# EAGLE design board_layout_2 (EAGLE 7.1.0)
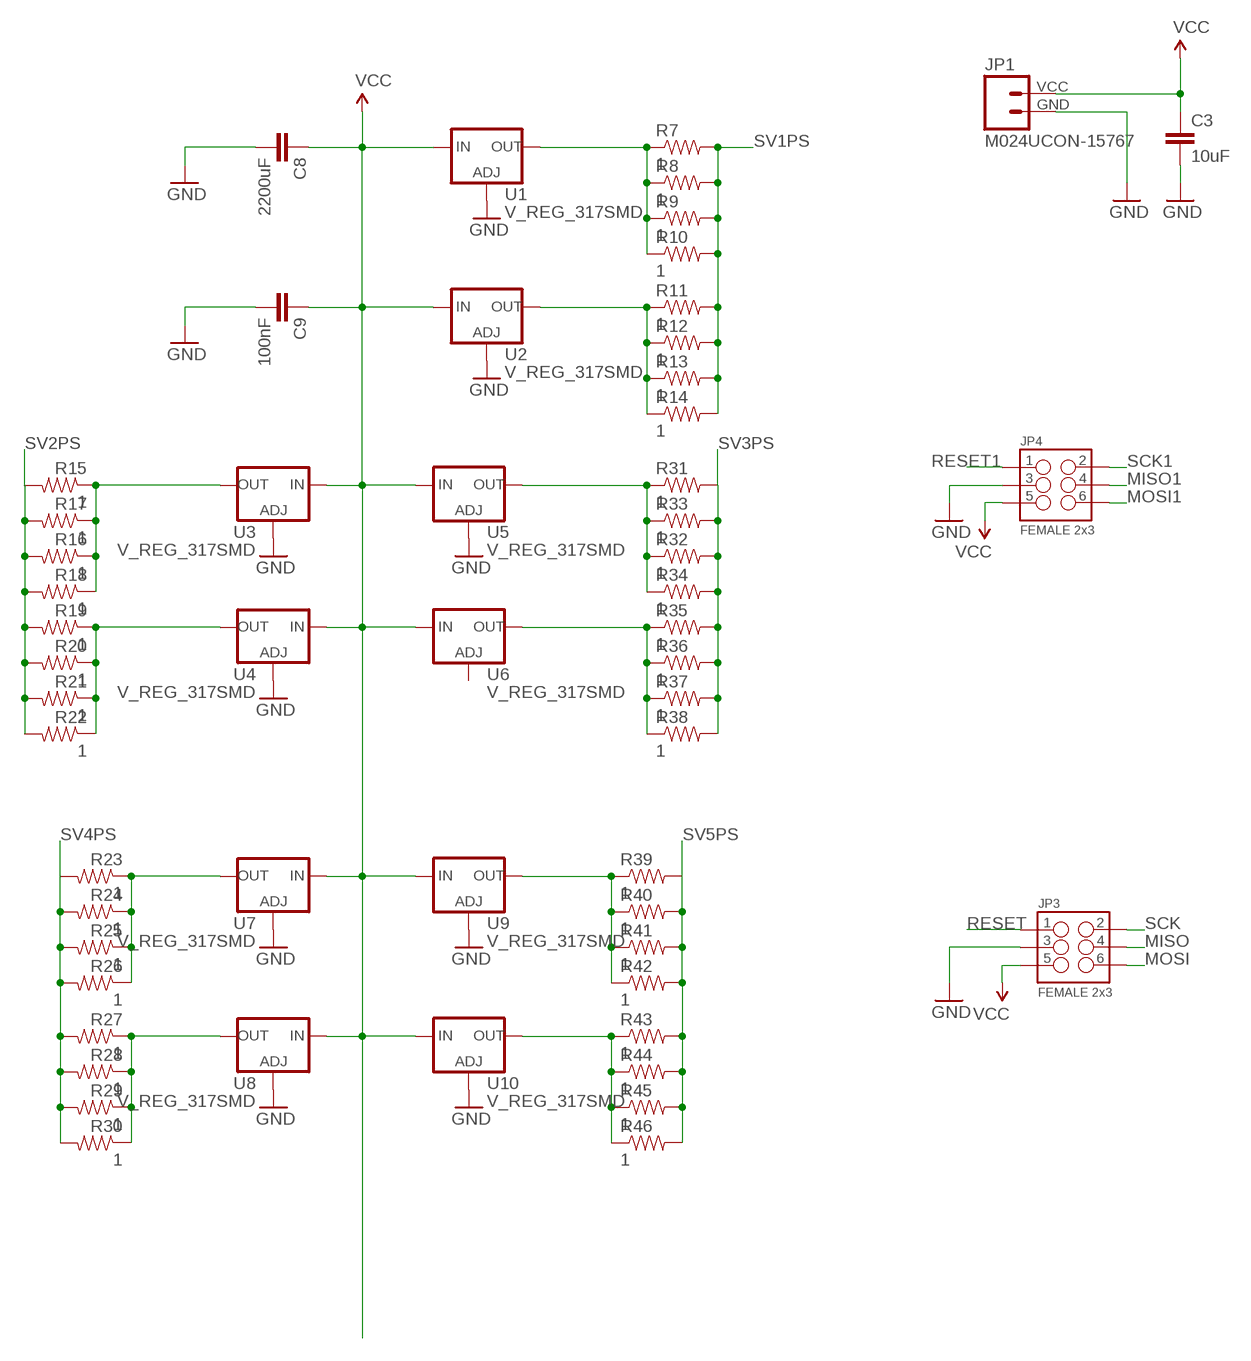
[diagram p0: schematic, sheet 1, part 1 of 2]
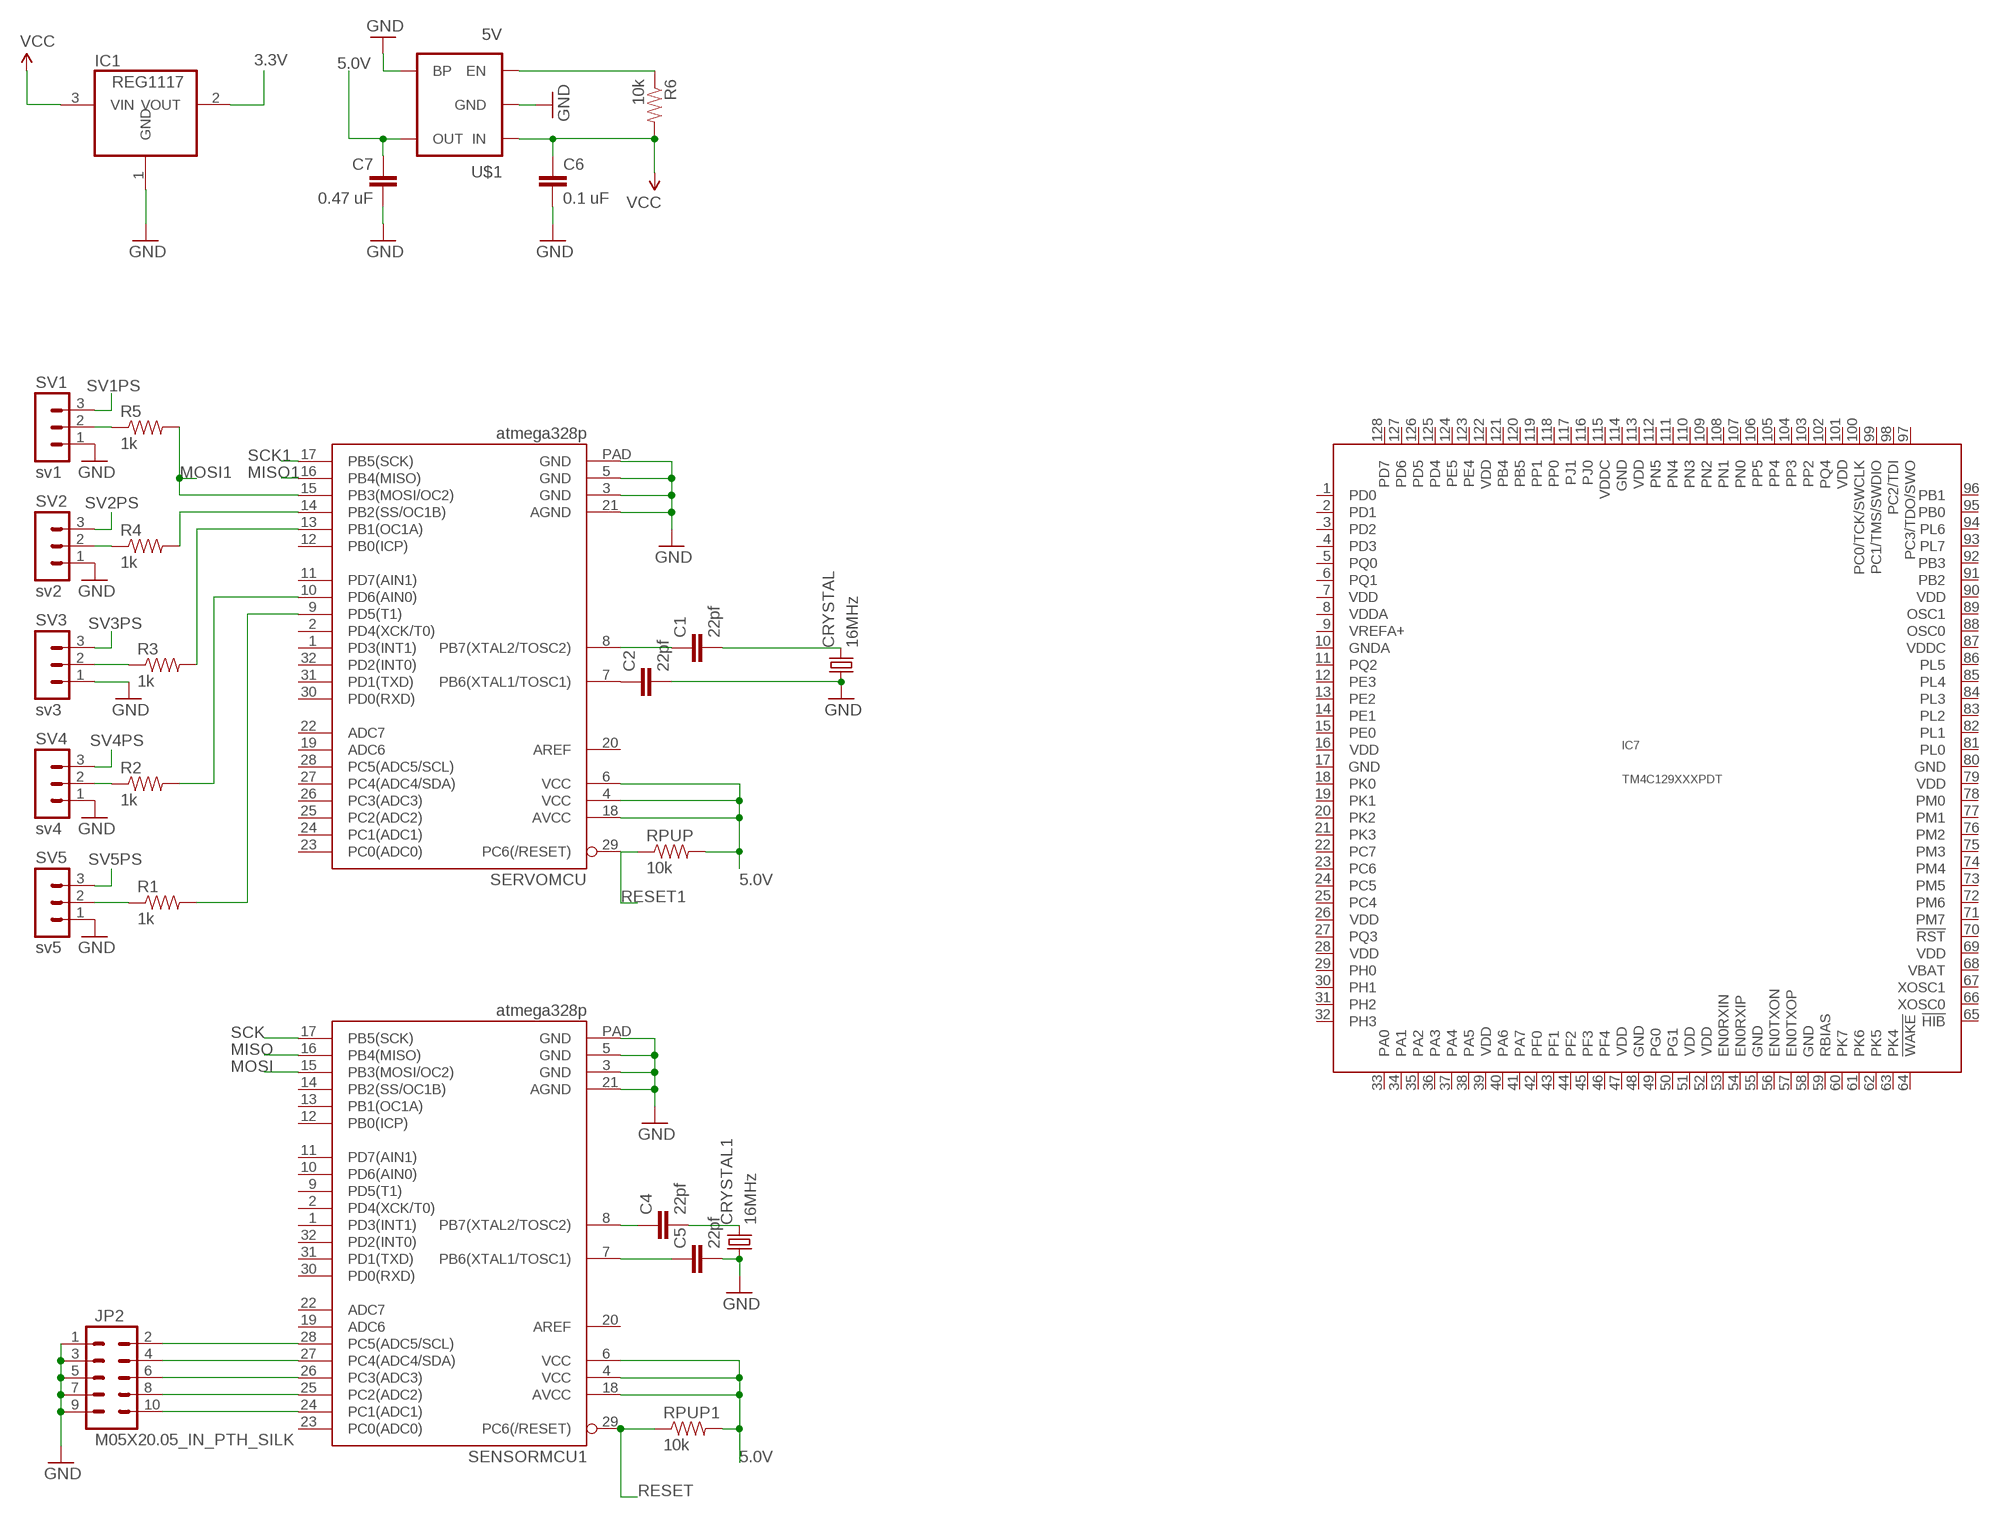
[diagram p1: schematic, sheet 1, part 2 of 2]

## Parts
C1  22pf  CAP0402-CAP  [0402-CAP]
C2  22pf  CAP0402-CAP  [0402-CAP]
C3  10uF  CAP0805  [0805]
C4  22pf  CAP0402-CAP  [0402-CAP]
C5  22pf  CAP0402-CAP  [0402-CAP]
C6  0.1 uF  CAP0805  [0805]
C7  0.47 uF  CAP0805  [0805]
C8  2200uF  CAP0805  [0805]
C9  100nF  CAP0805  [0805]
CRYSTAL  16MHz  CRYSTALTC26V  [TC26V]
CRYSTAL1  16MHz  CRYSTALTC26V  [TC26V]
IC1  REG1117  [SOT223]
IC7  TM4C129XXXPDT  [PDT_S-PQFP-G128]
JP1  M024UCON-15767  [JST-2-SMD-VERT]
JP2  M05X20.05_IN_PTH_SILK  [2X5_PTH_SILK_.05]
JP3  FEMALE 2x3  M03X2FEMALE  [2X3]
JP4  FEMALE 2x3  M03X2FEMALE  [2X3]
R1  1k  RESISTOR0402-RES  [0402-RES]
R2  1k  RESISTOR0402-RES  [0402-RES]
R3  1k  RESISTOR0402-RES  [0402-RES]
R4  1k  RESISTOR0402-RES  [0402-RES]
R5  1k  RESISTOR0402-RES  [0402-RES]
R6  10k  RESISTOR0805-RES  [0805]
R7  1  RESISTOR0805-RES  [0805]
R8  1  RESISTOR0805-RES  [0805]
R9  1  RESISTOR0805-RES  [0805]
R10  1  RESISTOR0805-RES  [0805]
R11  1  RESISTOR0805-RES  [0805]
R12  1  RESISTOR0805-RES  [0805]
R13  1  RESISTOR0805-RES  [0805]
R14  1  RESISTOR0805-RES  [0805]
R15  1  RESISTOR0805-RES  [0805]
R16  1  RESISTOR0805-RES  [0805]
R17  1  RESISTOR0805-RES  [0805]
R18  1  RESISTOR0805-RES  [0805]
R19  1  RESISTOR0805-RES  [0805]
R20  1  RESISTOR0805-RES  [0805]
R21  1  RESISTOR0805-RES  [0805]
R22  1  RESISTOR0805-RES  [0805]
R23  1  RESISTOR0805-RES  [0805]
R24  1  RESISTOR0805-RES  [0805]
R25  1  RESISTOR0805-RES  [0805]
R26  1  RESISTOR0805-RES  [0805]
R27  1  RESISTOR0805-RES  [0805]
R28  1  RESISTOR0805-RES  [0805]
R29  1  RESISTOR0805-RES  [0805]
R30  1  RESISTOR0805-RES  [0805]
R31  1  RESISTOR0805-RES  [0805]
R32  1  RESISTOR0805-RES  [0805]
R33  1  RESISTOR0805-RES  [0805]
R34  1  RESISTOR0805-RES  [0805]
R35  1  RESISTOR0805-RES  [0805]
R36  1  RESISTOR0805-RES  [0805]
R37  1  RESISTOR0805-RES  [0805]
R38  1  RESISTOR0805-RES  [0805]
R39  1  RESISTOR0805-RES  [0805]
R40  1  RESISTOR0805-RES  [0805]
R41  1  RESISTOR0805-RES  [0805]
R42  1  RESISTOR0805-RES  [0805]
R43  1  RESISTOR0805-RES  [0805]
R44  1  RESISTOR0805-RES  [0805]
R45  1  RESISTOR0805-RES  [0805]
R46  1  RESISTOR0805-RES  [0805]
RPUP  10k  RESISTOR0402-RES  [0402-RES]
RPUP1  10k  RESISTOR0402-RES  [0402-RES]
SENSORMCU1  atmega328p  ATMEGA328P_MLFMLF32  [MLF32-PAD]
SERVOMCU  atmega328p  ATMEGA328P_MLFMLF32  [MLF32-PAD]
SV1  sv1  MA03-1  [MA03-1]
SV2  sv2  MA03-1  [MA03-1]
SV3  sv3  MA03-1  [MA03-1]
SV4  sv4  MA03-1  [MA03-1]
SV5  sv5  MA03-1  [MA03-1]
U1  V_REG_317SMD  [SOT223]
U2  V_REG_317SMD  [SOT223]
U3  V_REG_317SMD  [SOT223]
U4  V_REG_317SMD  [SOT223]
U5  V_REG_317SMD  [SOT223]
U6  V_REG_317SMD  [SOT223]
U7  V_REG_317SMD  [SOT223]
U8  V_REG_317SMD  [SOT223]
U9  V_REG_317SMD  [SOT223]
U10  V_REG_317SMD  [SOT223]
U$1  5V  V_REG_MIC52055V  [SOT23-5]

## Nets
3.3V: IC1.2(VOUT)
5.0V: C7.1 RPUP1.2 RPUP.2 SENSORMCU1.4(VCC) SENSORMCU1.6(VCC) SENSORMCU1.18(AVCC) SERVOMCU.4(VCC) SERVOMCU.6(VCC) SERVOMCU.18(AVCC) U$1.5(OUT)
GND: C2.2 C3.2 C5.2 C6.2 C7.2 C8.2 C9.2 CRYSTAL1.1 CRYSTAL.1 IC1.1(GND) JP1.GND JP2.1 JP2.3 JP2.5 JP2.7 JP2.9 JP3.3 JP4.3 SENSORMCU1.3(GND) SENSORMCU1.5(GND) SENSORMCU1.21(AGND) SENSORMCU1.PAD(GND) SERVOMCU.3(GND) SERVOMCU.5(GND) SERVOMCU.21(AGND) SERVOMCU.PAD(GND) SV1.1 SV2.1 SV3.1 SV4.1 SV5.1 U1.1(ADJ) U2.1(ADJ) U3.1(ADJ) U4.1(ADJ) U5.1(ADJ) U7.1(ADJ) U8.1(ADJ) U9.1(ADJ) U10.1(ADJ) U$1.2(GND) U$1.4(BP)
MISO: JP3.4 SENSORMCU1.16(PB4(MISO))
MISO1: JP4.4 SERVOMCU.16(PB4(MISO))
MOSI: JP3.6 SENSORMCU1.15(PB3(MOSI/OC2))
MOSI1: JP4.6 R5.2 SERVOMCU.15(PB3(MOSI/OC2))
N$1: R6.1 U$1.3(EN)
N$2: R4.2 SERVOMCU.14(PB2(SS/OC1B))
N$3: R3.2 SERVOMCU.13(PB1(OC1A))
N$5: R2.1 SV4.2
N$6: R1.1 SV5.2
N$7: R2.2 SERVOMCU.10(PD6(AIN0))
N$8: R1.2 SERVOMCU.9(PD5(T1))
N$9: R3.1 SV3.2
N$10: C1.1 SERVOMCU.8(PB7(XTAL2/TOSC2))
N$11: C2.1 SERVOMCU.7(PB6(XTAL1/TOSC1))
N$12: R5.1 SV1.2
N$13: R4.1 SV2.2
N$14: R7.1 R8.1 R9.1 R10.1 U1.2(OUT)
N$15: JP2.10 SENSORMCU1.24(PC1(ADC1))
N$16: JP2.8 SENSORMCU1.25(PC2(ADC2))
N$17: C4.1 SENSORMCU1.8(PB7(XTAL2/TOSC2))
N$18: C4.2 CRYSTAL1.2
N$19: C5.1 SENSORMCU1.7(PB6(XTAL1/TOSC1))
N$20: C1.2 CRYSTAL.2
N$21: JP2.6 SENSORMCU1.26(PC3(ADC3))
N$22: JP2.4 SENSORMCU1.27(PC4(ADC4/SDA))
N$23: JP2.2 SENSORMCU1.28(PC5(ADC5/SCL))
N$24: R23.1 R24.1 R25.1 R26.1 U7.2(OUT)
N$27: R27.1 R28.1 R29.1 R30.1 U8.2(OUT)
N$28: R35.1 R36.1 R37.1 R38.1 U6.2(OUT)
N$29: R39.1 R40.1 R41.1 R42.1 U9.2(OUT)
N$31: R43.1 R44.1 R45.1 R46.1 U10.2(OUT)
N$140: R11.1 R12.1 R13.1 R14.1 U2.2(OUT)
N$1111: R15.1 R16.1 R17.1 R18.1 U3.2(OUT)
N$10101: R31.1 R32.1 R33.1 R34.1 U5.2(OUT)
NET$1300: R19.1 R20.1 R21.1 R22.1 U4.2(OUT)
RESET: JP3.1 RPUP1.1 SENSORMCU1.29(PC6(/RESET))
RESET1: JP4.1 RPUP.1 SERVOMCU.29(PC6(/RESET))
SCK: JP3.2 SENSORMCU1.17(PB5(SCK))
SCK1: JP4.2 SERVOMCU.17(PB5(SCK))
SV1PS: R7.2 R8.2 R9.2 R10.2 R11.2 R12.2 R13.2 R14.2 SV1.3
SV2PS: R15.2 R16.2 R17.2 R18.2 R19.2 R20.2 R21.2 R22.2 SV2.3
SV3PS: R31.2 R32.2 R33.2 R34.2 R35.2 R36.2 R37.2 R38.2 SV3.3
SV4PS: R23.2 R24.2 R25.2 R26.2 R27.2 R28.2 R29.2 R30.2 SV4.3
SV5PS: R39.2 R40.2 R41.2 R42.2 R43.2 R44.2 R45.2 R46.2 SV5.3
VCC: C3.1 C6.1 C8.1 C9.1 IC1.3(VIN) JP1.VCC JP3.5 JP4.5 R6.2 U1.3(IN) U2.3(IN) U3.3(IN) U4.3(IN) U5.3(IN) U6.3(IN) U7.3(IN) U8.3(IN) U9.3(IN) U10.3(IN) U$1.1(IN)
Unconnected: IC7.1(PD0) IC7.2(PD1) IC7.3(PD2) IC7.4(PD3) IC7.5(PQ0) IC7.6(PQ1) IC7.7(VDD) IC7.8(VDDA) IC7.9(VREFA+) IC7.10(GNDA) IC7.11(PQ2) IC7.12(PE3) IC7.13(PE2) IC7.14(PE1) IC7.15(PE0) IC7.16(VDD) IC7.17(GND) IC7.18(PK0) IC7.19(PK1) IC7.20(PK2) IC7.21(PK3) IC7.22(PC7) IC7.23(PC6) IC7.24(PC5) IC7.25(PC4) IC7.26(VDD) IC7.27(PQ3) IC7.28(VDD) IC7.29(PH0) IC7.30(PH1) IC7.31(PH2) IC7.32(PH3) IC7.33(PA0) IC7.34(PA1) IC7.35(PA2) IC7.36(PA3) IC7.37(PA4) IC7.38(PA5) IC7.39(VDD) IC7.40(PA6) IC7.41(PA7) IC7.42(PF0) IC7.43(PF1) IC7.44(PF2) IC7.45(PF3) IC7.46(PF4) IC7.47(VDD) IC7.48(GND) IC7.49(PG0) IC7.50(PG1) IC7.51(VDD) IC7.52(VDD) IC7.53(EN0RXIN) IC7.54(EN0RXIP) IC7.55(GND) IC7.56(EN0TXON) IC7.57(EN0TXOP) IC7.58(GND) IC7.59(RBIAS) IC7.60(PK7) IC7.61(PK6) IC7.62(PK5) IC7.63(PK4) IC7.64(!WAKE) IC7.65(!HIB) IC7.66(XOSC0) IC7.67(XOSC1) IC7.68(VBAT) IC7.69(VDD) IC7.70(!RST) IC7.71(PM7) IC7.72(PM6) IC7.73(PM5) IC7.74(PM4) IC7.75(PM3) IC7.76(PM2) IC7.77(PM1) IC7.78(PM0) IC7.79(VDD) IC7.80(GND) IC7.81(PL0) IC7.82(PL1) IC7.83(PL2) IC7.84(PL3) IC7.85(PL4) IC7.86(PL5) IC7.87(VDDC) IC7.88(OSC0) IC7.89(OSC1) IC7.90(VDD) IC7.91(PB2) IC7.92(PB3) IC7.93(PL7) IC7.94(PL6) IC7.95(PB0) IC7.96(PB1) IC7.97(PC3/TDO/SWO) IC7.98(PC2/TDI) IC7.99(PC1/TMS/SWDIO) IC7.100(PC0/TCK/SWCLK) IC7.101(VDD) IC7.102(PQ4) IC7.103(PP2) IC7.104(PP3) IC7.105(PP4) IC7.106(PP5) IC7.107(PN0) IC7.108(PN1) IC7.109(PN2) IC7.110(PN3) IC7.111(PN4) IC7.112(PN5) IC7.113(VDD) IC7.114(GND) IC7.115(VDDC) IC7.116(PJ0) IC7.117(PJ1) IC7.118(PP0) IC7.119(PP1) IC7.120(PB5) IC7.121(PB4) IC7.122(VDD) IC7.123(PE4) IC7.124(PE5) IC7.125(PD4) IC7.126(PD5) IC7.127(PD6) IC7.128(PD7) SENSORMCU1.1(PD3(INT1)) SENSORMCU1.2(PD4(XCK/T0)) SENSORMCU1.9(PD5(T1)) SENSORMCU1.10(PD6(AIN0)) SENSORMCU1.11(PD7(AIN1)) SENSORMCU1.12(PB0(ICP)) SENSORMCU1.13(PB1(OC1A)) SENSORMCU1.14(PB2(SS/OC1B)) SENSORMCU1.19(ADC6) SENSORMCU1.20(AREF) SENSORMCU1.22(ADC7) SENSORMCU1.23(PC0(ADC0)) SENSORMCU1.30(PD0(RXD)) SENSORMCU1.31(PD1(TXD)) SENSORMCU1.32(PD2(INT0)) SERVOMCU.1(PD3(INT1)) SERVOMCU.2(PD4(XCK/T0)) SERVOMCU.11(PD7(AIN1)) SERVOMCU.12(PB0(ICP)) SERVOMCU.19(ADC6) SERVOMCU.20(AREF) SERVOMCU.22(ADC7) SERVOMCU.23(PC0(ADC0)) SERVOMCU.24(PC1(ADC1)) SERVOMCU.25(PC2(ADC2)) SERVOMCU.26(PC3(ADC3)) SERVOMCU.27(PC4(ADC4/SDA)) SERVOMCU.28(PC5(ADC5/SCL)) SERVOMCU.30(PD0(RXD)) SERVOMCU.31(PD1(TXD)) SERVOMCU.32(PD2(INT0)) U6.1(ADJ)

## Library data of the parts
C1 C2 C4-C7 = SparkFun-Passives:CAP: Capacitor
C3 C8 C9 = SparkFun-Capacitors:CAP: Capacitor
CRYSTAL CRYSTAL1 = crystal:CRYSTAL: CRYSTAL; OC_FARNELL: unknown; OC_NEWARK: unknown
IC1 = burr-brown:REG1117: 800mA and 1A Low Dropout (LDO) Positive Regulator 1.8V, 2.5V, 2.85V, 3.3V, 5V, and Adj; MPN: REG1117; OC_FARNELL: 1097566; OC_NEWARK: 14P6981
IC7 = ti-tiva:TM4C129XXX
JP1 = SparkFun-Connectors:M02: Standard 2-pin 0.1" header. Use with
JP2 = SparkFun-Connectors:M05X2: Header 5x2 Standard 10-pin dual row 0.1" header. Commonly used with AVR-ISP. Use with Spark Fun Electronics SKU: PRT-00778
JP3 JP4 = SparkFun-Connectors:M03X2: 2x3 .1" header. Shrouded, with keying- CONN-10681 SMT- CONN-11415 Pogo pins- HW-11044; PROD_ID: CONN-11566
R1-R46 RPUP RPUP1 = SparkFun-Passives:RESISTOR: Resistor
SENSORMCU1 SERVOMCU = SparkFun-DigitalIC:ATMEGA328P_MLF: 32-Pin Atmega328 part Commonly used on Arduino compatible boards Available in QFP and QFN packages TQFP is IC-09069 QFN is non-stock
SV1-SV5 = con-lstb:MA03-1: PIN HEADER; OC_FARNELL: unknown; OC_NEWARK: unknown
U1-U10 = SparkFun-PowerIC:V_REG_317: Voltage Regulator Standard LM317 adjustable voltage regulator. AOI (Adjust Output Input). Google 'LM317 Calculator' for easy to use app to get the two resistor values needed. 240/720 for 5V output. 240/390 for 3.3V output. Spark Fun Electronics SKU : COM-00527
U$1 = SparkFun-PowerIC:V_REG_MIC5205: V_REG MIC5219 Standard 3.3V and 5V 150mA LDO voltage regulator in SOT-23 layout. Micrel part MIC5205. BP (by-pass) pin is used to lower output noise with 470pF cap, may be left open.; PROD_ID: VREG-00823

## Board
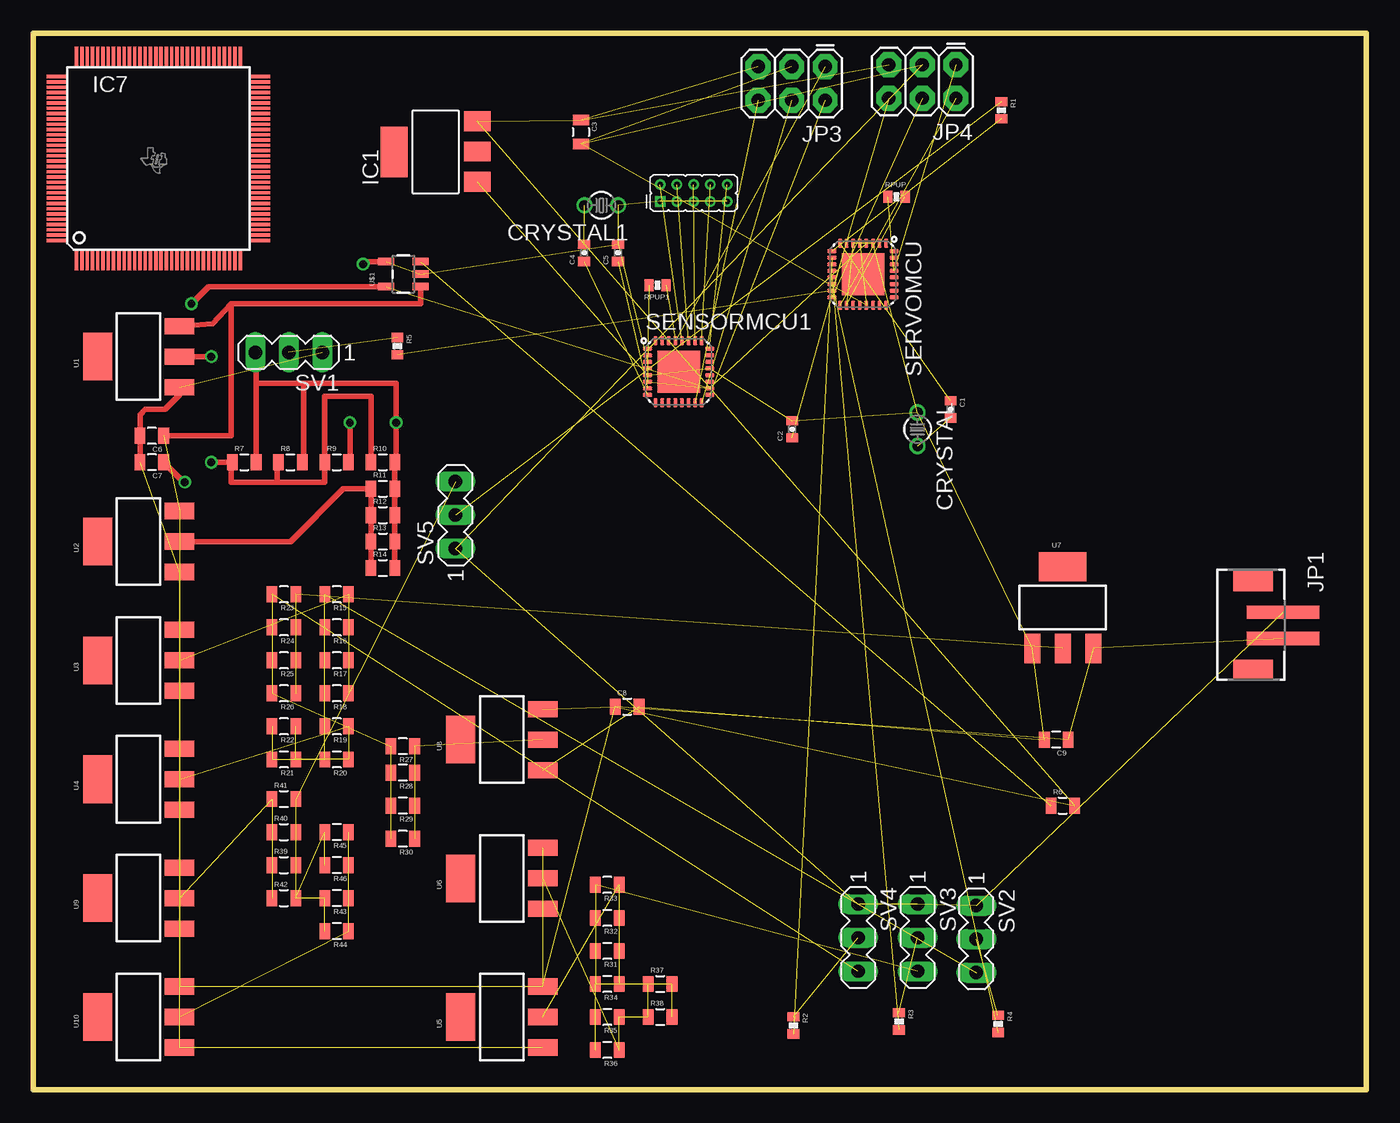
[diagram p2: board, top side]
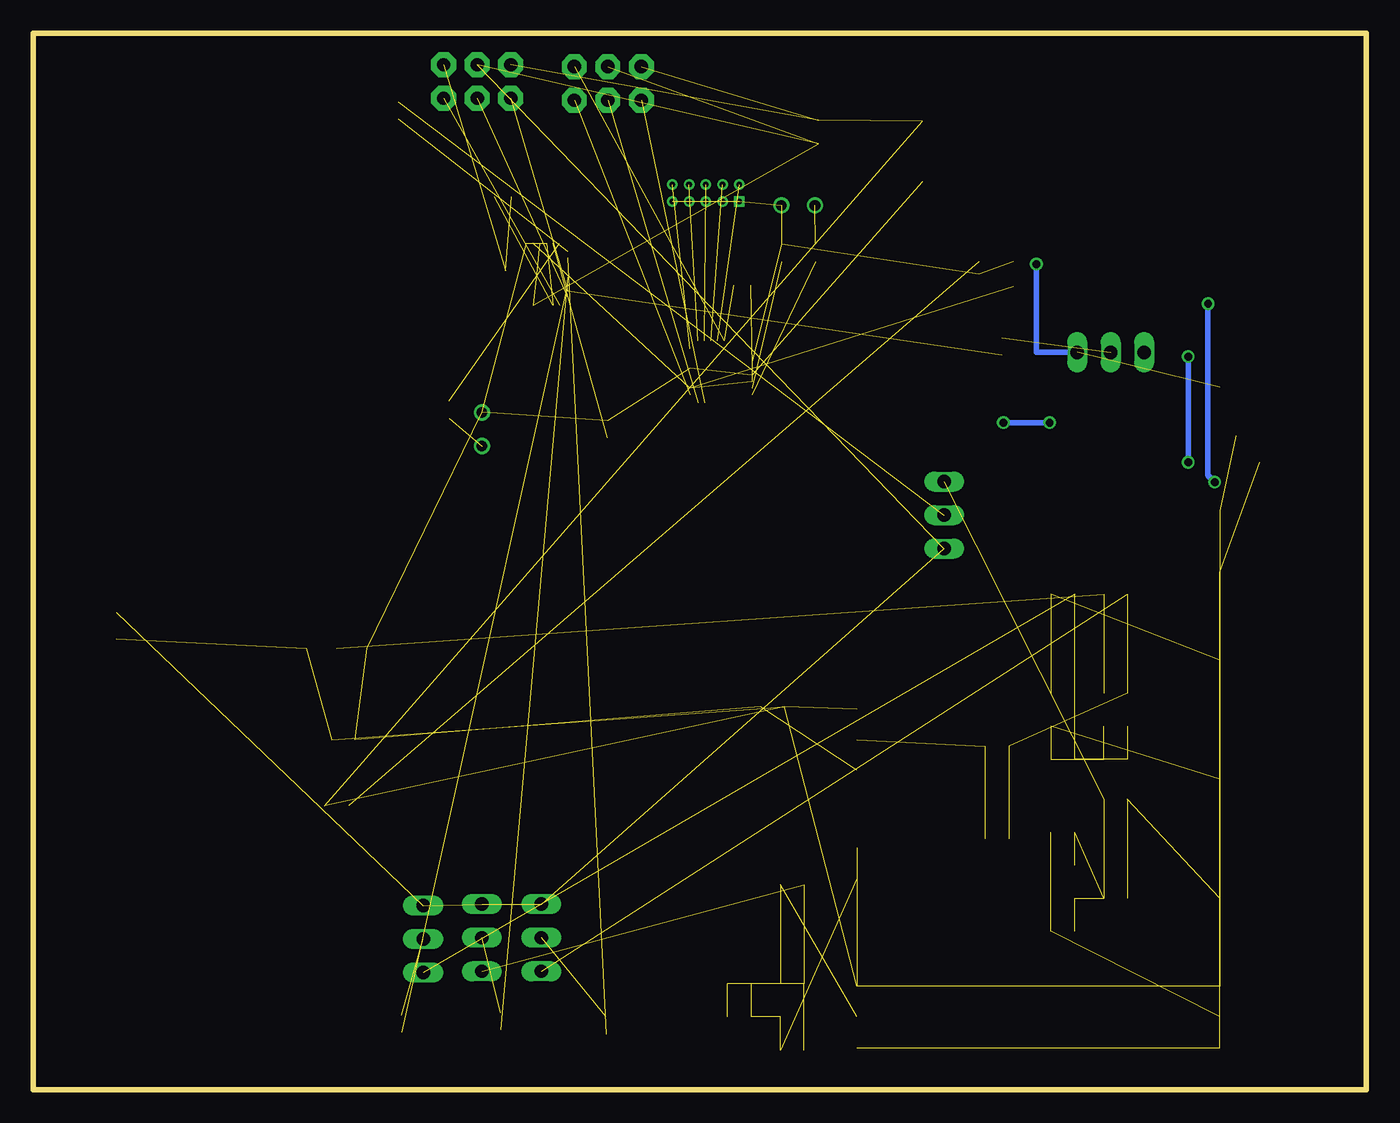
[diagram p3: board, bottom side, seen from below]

Size 101 x 80 mm. Coordinates in mm from the lower left corner, seen from the top.
Outline: 0,0 101,0 101,80 0,80 0,0
Copper layers (1*16): Top 0.0356mm / dielectric 1.5011mm / Bottom 0.0356mm
Design rules "LaenPCBOrder": minimum track width 6mil, minimum drill 13mil, track to track 6mil, track to pad 6mil, pad to pad 6mil, via to via 6mil, smd to smd 6mil, copper to edge 15mil, drill to drill 6mil, minimum pad ring 7mil, minimum via ring 7mil, stop-mask expansion 3mil, vias tented up to drill 0mil, thermal gap 10mil

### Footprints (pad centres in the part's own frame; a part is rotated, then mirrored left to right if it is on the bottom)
0402-CAP = smd 0.7 x 0.9: 1 -0.65,0; 2 0.65,0
0805 = smd 0.8 x 1.2: 1 -0.9,0; 2 0.9,0
TC26V = drill 0.813: 1 -1.27,0; 2 1.27,0
SOT223 = smd 1.499 x 2.007: 1 -2.261,-3.15; 2 0.025,-3.15; 3 2.311,-3.15 | smd 3.81 x 2.007: 4 0,3.15
PDT_S-PQFP-G128 = smd 0.25 x 1.6: 1 -6.2,-7.65; 2 -5.8,-7.65; 3 -5.4,-7.65; 4 -5,-7.65; 5 -4.6,-7.65; 6 -4.2,-7.65; 7 -3.8,-7.65; 8 -3.4,-7.65; 9 -3,-7.65; 10 -2.6,-7.65; 11 -2.2,-7.65; 12 -1.8,-7.65; 13 -1.4,-7.65; 14 -1,-7.65; 15 -0.6,-7.65; 16 -0.2,-7.65; 17 0.2,-7.65; 18 0.6,-7.65; 19 1,-7.65; 20 1.4,-7.65; 21 1.8,-7.65; 22 2.2,-7.65; 23 2.6,-7.65; 24 3,-7.65; 25 3.4,-7.65; 26 3.8,-7.65; 27 4.2,-7.65; 28 4.6,-7.65; 29 5,-7.65; 30 5.4,-7.65; 31 5.8,-7.65; 32 6.2,-7.65; 65 6.2,7.65; 66 5.8,7.65; 67 5.4,7.65; 68 5,7.65; 69 4.6,7.65; 70 4.2,7.65; 71 3.8,7.65; 72 3.4,7.65; 73 3,7.65; 74 2.6,7.65; 75 2.2,7.65; 76 1.8,7.65; 77 1.4,7.65; 78 1,7.65; 79 0.6,7.65; 80 0.2,7.65; 81 -0.2,7.65; 82 -0.6,7.65; 83 -1,7.65; 84 -1.4,7.65; 85 -1.8,7.65; 86 -2.2,7.65; 87 -2.6,7.65; 88 -3,7.65; 89 -3.4,7.65; 90 -3.8,7.65; 91 -4.2,7.65; 92 -4.6,7.65; 93 -5,7.65; 94 -5.4,7.65; 95 -5.8,7.65; 96 -6.2,7.65 | smd 1.6 x 0.25: 33 7.65,-6.2; 34 7.65,-5.8; 35 7.65,-5.4; 36 7.65,-5; 37 7.65,-4.6; 38 7.65,-4.2; 39 7.65,-3.8; 40 7.65,-3.4; 41 7.65,-3; 42 7.65,-2.6; 43 7.65,-2.2; 44 7.65,-1.8; 45 7.65,-1.4; 46 7.65,-1; 47 7.65,-0.6; 48 7.65,-0.2; 49 7.65,0.2; 50 7.65,0.6; 51 7.65,1; 52 7.65,1.4; 53 7.65,1.8; 54 7.65,2.2; 55 7.65,2.6; 56 7.65,3; 57 7.65,3.4; 58 7.65,3.8; 59 7.65,4.2; 60 7.65,4.6; 61 7.65,5; 62 7.65,5.4; 63 7.65,5.8; 64 7.65,6.2; 97 -7.65,6.2; 98 -7.65,5.8; 99 -7.65,5.4; 100 -7.65,5; 101 -7.65,4.6; 102 -7.65,4.2; 103 -7.65,3.8; 104 -7.65,3.4; 105 -7.65,3; 106 -7.65,2.6; 107 -7.65,2.2; 108 -7.65,1.8; 109 -7.65,1.4; 110 -7.65,1; 111 -7.65,0.6; 112 -7.65,0.2; 113 -7.65,-0.2; 114 -7.65,-0.6; 115 -7.65,-1; 116 -7.65,-1.4; 117 -7.65,-1.8; 118 -7.65,-2.2; 119 -7.65,-2.6; 120 -7.65,-3; 121 -7.65,-3.4; 122 -7.65,-3.8; 123 -7.65,-4.2; 124 -7.65,-4.6; 125 -7.65,-5; 126 -7.65,-5.4; 127 -7.65,-5.8; 128 -7.65,-6.2
JST-2-SMD-VERT = smd 1 x 5.5: GND 1,-2; VCC -1,-2 | smd 1.6 x 3: P$1 -3.4,0.27; P$2 3.4,0.27
2X5_PTH_SILK_.05 = drill 0.432 square: 1 0,6.35 | drill 0.432: 2 1.27,6.35; 3 0,5.08; 4 1.27,5.08; 5 0,3.81; 6 1.27,3.81; 7 0,2.54; 8 1.27,2.54; 9 0,1.27; 10 1.27,1.27
2X3 = drill 1.016 pad 1.88 octagon: 1 0,0; 2 0,2.54; 3 2.54,0; 4 2.54,2.54; 5 5.08,0; 6 5.08,2.54
0402-RES = smd 0.7 x 0.9: 1 -0.65,0; 2 0.65,0
MLF32-PAD = smd 0.7 x 0.3: 1 -2.35,1.75; 2 -2.35,1.25; 3 -2.35,0.75; 4 -2.35,0.25; 5 -2.35,-0.25; 6 -2.35,-0.75; 7 -2.35,-1.25; 8 -2.35,-1.75; 17 2.35,-1.75; 18 2.35,-1.25; 19 2.35,-0.75; 20 2.35,-0.25; 21 2.35,0.25; 22 2.35,0.75; 23 2.35,1.25; 24 2.35,1.75 | smd 0.3 x 0.7: 9 -1.75,-2.35; 10 -1.25,-2.35; 11 -0.75,-2.35; 12 -0.25,-2.35; 13 0.25,-2.35; 14 0.75,-2.35; 15 1.25,-2.35; 16 1.75,-2.35; 25 1.75,2.35; 26 1.25,2.35; 27 0.75,2.35; 28 0.25,2.35; 29 -0.25,2.35; 30 -0.75,2.35; 31 -1.25,2.35; 32 -1.75,2.35 | smd 3.2 x 3.2: PAD 0,0
MA03-1 = drill 1.016 long: 1 -2.54,0; 2 0,0; 3 2.54,0
SOT223' = smd 1.219 x 2.235: 1 -2.311,-3.099; 2 0,-3.099; 3 2.311,-3.099 | smd 3.6 x 2.2: 4 0,3.099
SOT23-5 = smd 0.55 x 1.2: 1 -0.95,-1.3; 2 0,-1.3; 3 0.95,-1.3; 4 0.95,1.3; 5 -0.95,1.3

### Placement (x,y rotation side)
C1  69.5,51.5 270 top
C2  57.5,50 90 top
C3  41.5,72.5 270 top
C4  41.75,63.35 90 top
C5  44.3,63.35 90 top
C6  9,49.5 180 top
C7  9,47.5 180 top
C8  45,29 0 top
C9  77.5,26.5 180 top
CRYSTAL  67,50 270 top
CRYSTAL1  43.05,66.95 180 top
IC1  30.5,71 90 top
IC7  9.5,70.5 0 top
JP1  92.69,35.15 90 top
JP2  53.85,67.25 90 top
JP3  60,77.45 180 top
JP4  69.9,77.6 180 top
R1  73.35,74.15 270 top
R2  57.6,4.86 270 top
R3  65.6,5.17 270 top
R4  73.1,4.98 270 top
R5  27.6,56.29 270 top
R6  78,21.5 0 top
R7  16,47.5 0 top
R8  19.5,47.5 0 top
R9  23,47.5 0 top
R10  26.5,47.5 0 top
R11  26.5,45.5 0 top
R12  26.5,43.5 0 top
R13  26.5,41.5 0 top
R14  26.5,39.5 0 top
R15  23,37.5 180 top
R16  23,35 180 top
R17  23,32.5 180 top
R18  23,30 180 top
R19  23,27.5 180 top
R20  23,25 180 top
R21  19,25 180 top
R22  19,27.5 180 top
R23  19,37.5 180 top
R24  19,35 180 top
R25  19,32.5 180 top
R26  19,30 180 top
R27  28,26 180 top
R28  28,24 180 top
R29  28,21.5 180 top
R30  28,19 180 top
R31  43.5,10.5 180 top
R32  43.5,13 180 top
R33  43.5,15.5 180 top
R34  43.5,8 180 top
R35  43.5,5.5 180 top
R36  43.5,3 180 top
R37  47.5,8 0 top
R38  47.5,5.5 0 top
R39  19,17 0 top
R40  19,19.5 0 top
R41  19,22 0 top
R42  19,14.5 0 top
R43  23,14.5 180 top
R44  23,12 180 top
R45  23,19.5 180 top
R46  23,17 180 top
RPUP  65.4,67.6 0 top
RPUP1  47.3,60.9 180 top
SENSORMCU1  48.9,54.35 0 top
SERVOMCU  62.87,61.74 270 top
SV1  19.37,55.83 180 top
SV2  71.45,11.4 270 top
SV3  67,11.5 270 top
SV4  62.5,11.5 270 top
SV5  32,43.5 90 top
U1  V_REG_317SMD  [SOT223']  8,55.5 90 top
U2  V_REG_317SMD  [SOT223']  8,41.5 90 top
U3  V_REG_317SMD  [SOT223']  8,32.5 90 top
U4  V_REG_317SMD  [SOT223']  8,23.5 90 top
U5  V_REG_317SMD  [SOT223']  35.5,5.5 90 top
U6  V_REG_317SMD  [SOT223']  35.5,16 90 top
U7  V_REG_317SMD  [SOT223']  78,36.5 0 top
U8  V_REG_317SMD  [SOT223']  35.5,26.5 90 top
U9  V_REG_317SMD  [SOT223']  8,14.5 90 top
U10  V_REG_317SMD  [SOT223']  8,5.5 90 top
U$1  28.05,61.75 90 top

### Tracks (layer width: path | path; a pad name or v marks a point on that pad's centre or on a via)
5.0V  (via drill 0.6)  (8 unrouted)
  Top 0.406: C7.1 11.4,46 v11.5,46 | v12,59.5 13.3,60.8 U$1.5
  Bottom 0.406: v11.5,46 12,46.5 v12,59.5
GND  (via drill 0.6)  (38 unrouted)
  Top 0.406: U1.1 11.1,52.6 10,51.5 8.5,51.5 8.1,51.1 C6.2 C7.2 | U$1.4 25,62.7 v25,62.5
  Bottom 0.406: v25,62.5 25,55.83 SV1.1
MISO  (1 unrouted)
MISO1  (1 unrouted)
MOSI  (1 unrouted)
MOSI1  (2 unrouted)
N$1  (1 unrouted)
N$2  (1 unrouted)
N$3  (1 unrouted)
N$5  (1 unrouted)
N$6  (1 unrouted)
N$7  (1 unrouted)
N$8  (1 unrouted)
N$9  (1 unrouted)
N$10  (1 unrouted)
N$11  (1 unrouted)
N$12  (1 unrouted)
N$13  (1 unrouted)
N$14  (via drill 0.6)
  Top 0.406: R8.1 18.5,47.5 18.5,46 | 18.5,46 15,46 15,47.5 | 15,47.5 R7.1 | 18.5,46 22.1,46 R9.1 22.1,52.5 25.6,52.5 R10.1 | 15,47.5 v13.5,47.5 | v13.5,55.5 U1.2
  Bottom 0.406: v13.5,47.5 v13.5,55.5
N$15  (1 unrouted)
N$16  (1 unrouted)
N$17  (1 unrouted)
N$18  (1 unrouted)
N$19  (1 unrouted)
N$20  (1 unrouted)
N$21  (1 unrouted)
N$22  (1 unrouted)
N$23  (1 unrouted)
N$24  (4 unrouted)
N$27  (4 unrouted)
N$28  (4 unrouted)
N$29  (4 unrouted)
N$31  (4 unrouted)
N$140
  Top 0.406: U2.2 19.5,41.5 23.5,45.5 R11.1 R12.1 R13.1 25.6,39.6 25.5,39.5 R14.1
N$1111  (4 unrouted)
N$10101  (4 unrouted)
NET$1300  (4 unrouted)
RESET  (2 unrouted)
RESET1  (2 unrouted)
SCK  (1 unrouted)
SCK1  (1 unrouted)
SV1PS  (via drill 0.6)
  Top 0.406: SV1.3 16.9,55.83 16.9,53.5 | 16.9,53.5 R7.2 | R14.2 R13.2 R12.2 27.4,44.9 27.5,45 27.5,45.4 R11.2 R10.2 27.5,47.6 v27.5,50.5 27.5,53.5 20.5,53.5 | 20.5,53.5 16.9,53.5 | R8.2 20.5,47.5 20.5,53.5 | R9.2 24,47.5 v24,50.5
  Bottom 0.406: v24,50.5 v27.5,50.5
SV2PS  (8 unrouted)
SV3PS  (8 unrouted)
SV4PS  (8 unrouted)
SV5PS  (8 unrouted)
VCC  (17 unrouted)
  Top 0.406: U1.3 13.6,58 15,59.5 | 15,59.5 15,49.5 C6.1 | 15,59.5 29.35,59.5 U$1.1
